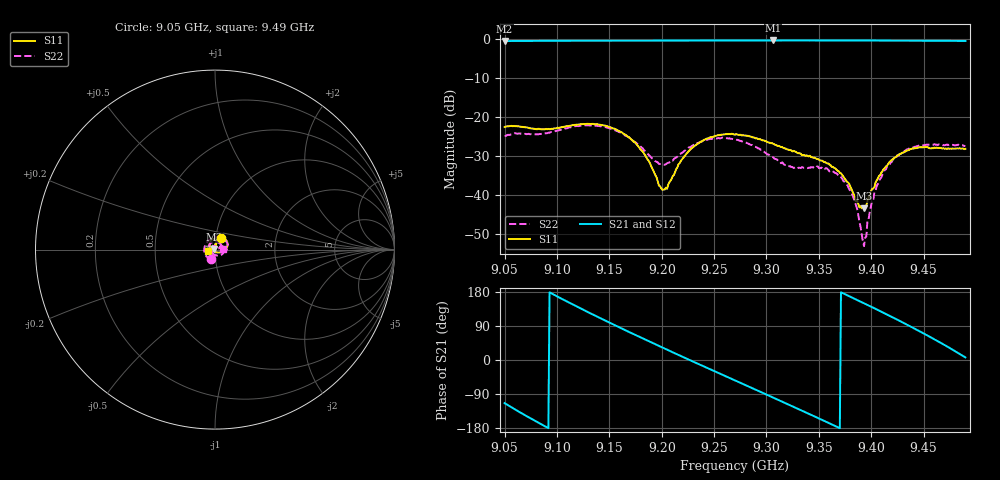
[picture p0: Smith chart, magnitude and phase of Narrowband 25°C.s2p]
!Agilent Technologies,N5230C,MY49001174,A.09.42.22
!Agilent N5230C: A.09.42.22
!Date: Friday, February 13, 2026 11:19:37
!Correction: S11(Full 2 Port(1,2))
!S21(Full 2 Port(1,2))
!S12(Full 2 Port(1,2))
!S22(Full 2 Port(1,2))
!S2P File: Measurements: S11, S21, S12, S22:
# Hz S  dB  R 50
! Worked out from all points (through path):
!   401 points, 9.05 GHz to 9.49 GHz, reference 50 ohm
!   highest |S21| = -0.42 dB at 9.3063 GHz (marker M1); lowest = -0.6 dB at 9.05 GHz (marker M2)
!   lowest |S11| = -43.5 dB at 9.3932 GHz (marker M3), VSWR 1.01, Z = 49.4 + j0.297 ohm
!   |S11| at or under -10 dB: start of sweep to end of sweep
!   |S22| runs from -53.2 to -22.1 dB; largest |S21 - S12| = 0.0023
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9.05e9  -22.62 61.7  -0.57 -113.8  -0.56 -113.8  -24.94 -110.3
9.0698e9  -22.70 55.6  -0.53 -146.3  -0.53 -146.3  -24.39 -168.8
9.0863e9  -23.22 55.1  -0.52 -171.7  -0.51 -171.7  -24.34 139.5
9.1039e9  -22.69 54.5  -0.50 162.4  -0.50 162.4  -23.32 90.4
9.1237e9  -21.91 44.5  -0.49 134.4  -0.49 134.4  -22.21 49.0
9.16e9  -23.75 7.7  -0.47 85.5  -0.46 85.4  -23.97 -2.3
9.1831e9  -29.47 -27.2  -0.44 55.4  -0.44 55.3  -28.59 -16.9
9.1974e9  -37.67 -76.6  -0.44 37.0  -0.44 37.0  -32.09 -0.4
9.204e9  -38.17 -134.6  -0.43 28.6  -0.44 28.6  -32.16 14.1
9.2326e9  -27.30 133.7  -0.43 -7.4  -0.44 -7.4  -26.84 25.1
9.27e9  -24.62 95.3  -0.44 -53.9  -0.44 -53.9  -25.84 -18.5
9.3063e9  -26.89 78.0  -0.42 -99.0  -0.43 -99.0  -30.34 -92.2
9.3437e9  -30.39 81.5  -0.43 -146.0  -0.43 -146.0  -32.96 146.5
9.3756e9  -36.16 83.4  -0.44 173.0  -0.44 173.0  -37.12 75.5
9.3844e9  -40.27 99.5  -0.44 161.4  -0.44 161.4  -41.84 52.8
9.3932e9  -43.52 153.2  -0.45 149.8  -0.45 149.7  -53.20 -35.9
9.4053e9  -36.30 -169.1  -0.46 133.4  -0.46 133.5  -37.75 -138.3
9.4174e9  -31.61 -164.8  -0.46 116.9  -0.46 116.9  -32.54 -166.0
9.435e9  -28.61 -170.9  -0.47 92.2  -0.48 92.1  -28.36 157.2
9.4526e9  -27.78 -175.9  -0.50 66.4  -0.50 66.4  -27.15 113.7
9.4735e9  -28.09 -169.3  -0.52 34.1  -0.51 34.1  -27.27 52.0
9.49e9  -28.24 -170.4  -0.55 6.8  -0.55 6.9  -27.56 3.7
